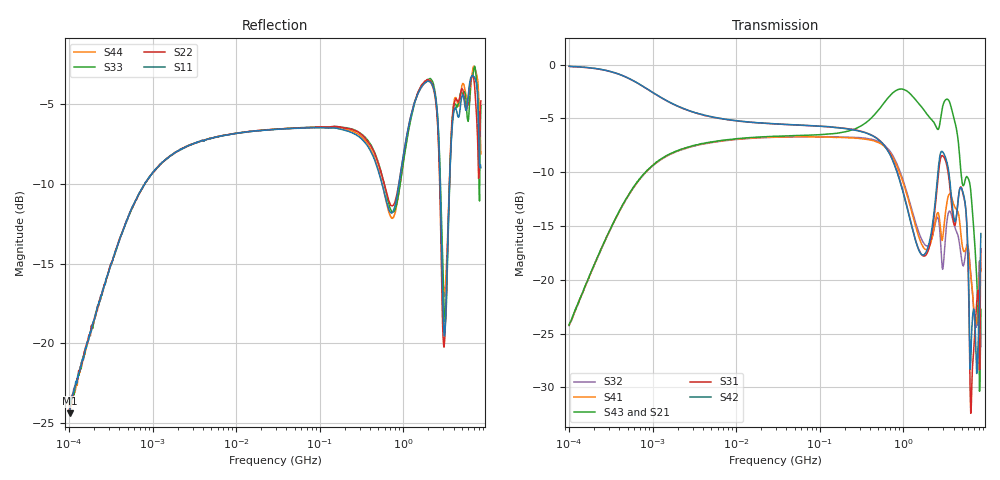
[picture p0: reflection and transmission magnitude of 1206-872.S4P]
!Agilent Technologies,E5071C,MY46110495,A.10.06
!Date: Tue Jun 06 12:42:36 2017
!Data & Calibration Information:
!Freq	S11:SOLT4(ON)	S12:SOLT4(ON)	S13:SOLT4(ON)	S14:SOLT4(ON)
!	S21:SOLT4(ON)	S22:SOLT4(ON)	S23:SOLT4(ON)	S24:SOLT4(ON)
!	S31:SOLT4(ON)	S32:SOLT4(ON)	S33:SOLT4(ON)	S34:SOLT4(ON)
!	S41:SOLT4(ON)	S42:SOLT4(ON)	S43:SOLT4(ON)	S44:SOLT4(ON)
!PortZ  Port1:50+j0  Port2:50+j0  Port3:50+j0  Port4:50+j0
!Above PortZ is port z conversion or system Z0 setting when saving the data.
!When reading, reference impedance value at option line is always used.
# Hz S dB R 50
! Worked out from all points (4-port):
!   801 points, 100 kHz to 8.5 GHz, reference 50 ohm
!   strongest paths, dB at 100 kHz, 1.721 MHz, 29.51 MHz, 502.3 MHz, 8.5 GHz:
!     S42: -0.2, -3.6, -5.5, -7.0, -15.7
!     S31: -0.2, -3.6, -5.5, -6.9, -17.1
!     S43: -24.2, -8.2, -6.7, -4.2, -22.7
!     S21: -24.3, -8.2, -6.7, -4.2, -22.8
!     S41: -24.2, -8.2, -6.7, -7.3, -19.2
!     S32: -24.3, -8.3, -6.7, -7.2, -26.2
!   lowest |S11| = -24.4 dB at 101.7 kHz (marker M1), VSWR 1.13, Z = 51.4 + j5.95 ohm
!   |S11| at or under -10 dB: start of sweep to 803.1 kHz; 557.3 MHz to 888.4 MHz (331.1 MHz wide, 45.8 % of centre); 2.764 GHz to 3.575 GHz (811.1 MHz wide, 25.6 % of centre)
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100000  -24.31 75.3  -24.25 79.5  -0.16 -3.3  -24.19 -100.8
        -24.28 79.2  -24.17 73.6  -24.25 -100.5  -0.18 -3.3
        -0.17 -3.4  -24.26 -100.7  -23.69 77.6  -24.28 79.3
        -24.20 -100.2  -0.15 -3.4  -24.21 79.0  -23.85 75.3
101665  -24.42 73.5  -24.07 80.1  -0.17 -3.4  -24.10 -101.0
        -24.10 79.6  -24.29 73.9  -24.11 -100.8  -0.18 -3.4
        -0.18 -3.4  -24.11 -100.7  -23.87 76.6  -24.02 79.4
        -24.09 -100.1  -0.15 -3.6  -23.99 79.1  -24.10 75.0
9.35121e8  -9.25 62.8  -2.41 -1.8  -11.02 -115.4  -10.34 63.1
           -2.42 -1.8  -9.21 59.8  -10.14 65.6  -11.15 -114.9
           -11.03 -115.5  -10.15 65.5  -9.72 60.3  -2.29 -1.2
           -10.34 63.2  -11.14 -114.8  -2.27 -1.2  -9.71 62.1
2.247738e9  -3.82 66.0  -5.28 -18.8  -15.26 154.5  -15.89 39.8
            -5.27 -18.7  -3.76 62.9  -15.87 33.5  -14.78 151.2
            -15.28 154.6  -15.89 33.6  -3.57 65.8  -5.25 -18.1
            -15.89 39.9  -14.77 151.1  -5.24 -18.1  -3.87 66.2
5.161627e9  -4.39 -83.2  -9.98 -49.5  -11.92 -8.0  -17.04 -177.6
            -10.01 -49.4  -4.07 -86.9  -18.64 168.1  -11.80 -6.3
            -11.94 -7.8  -18.66 168.5  -4.36 -87.2  -11.21 -49.3
            -17.09 -177.1  -11.81 -6.2  -11.21 -49.3  -3.69 -81.3
6.842542e9  -3.18 15.2  -15.21 -89.2  -27.41 23.4  -21.85 17.9
            -15.20 -89.0  -3.23 10.3  -21.89 6.9  -23.04 2.9
            -27.45 23.5  -21.85 7.3  -3.13 15.7  -14.36 -73.7
            -21.85 18.5  -23.03 2.8  -14.33 -73.4  -2.73 19.8
8.5e9  -8.97 117.7  -22.73 95.9  -17.12 63.8  -19.19 0.2
       -22.77 96.3  -4.78 124.5  -26.16 -15.4  -15.72 39.5
       -17.13 64.0  -26.19 -15.5  -5.09 130.3  -22.74 78.8
       -19.16 0.9  -15.70 40.0  -22.75 79.1  -8.11 103.2
